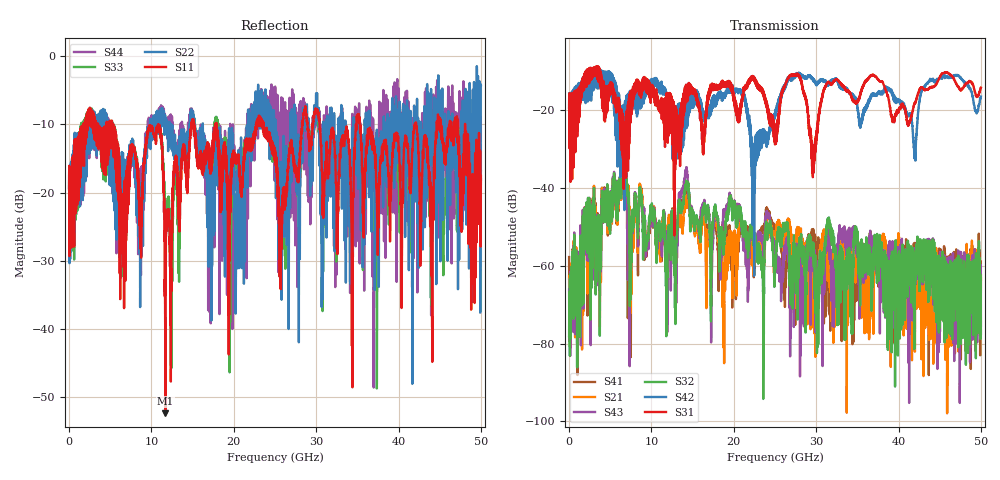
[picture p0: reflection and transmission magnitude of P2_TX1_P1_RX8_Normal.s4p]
!Keysight Technologies,N5225B,MY57041031,A.13.20.10
!Date: Friday, May 31, 2019 11:26:29
!Correction: S11(Full 4 Port(1,2,3,4))
!S12(Full 4 Port(1,2,3,4))
!S13(Full 4 Port(1,2,3,4))
!S14(Full 4 Port(1,2,3,4))
!S21(Full 4 Port(1,2,3,4))
!S22(Full 4 Port(1,2,3,4))
!S23(Full 4 Port(1,2,3,4))
!S24(Full 4 Port(1,2,3,4))
!S31(Full 4 Port(1,2,3,4))
!S32(Full 4 Port(1,2,3,4))
!S33(Full 4 Port(1,2,3,4))
!S34(Full 4 Port(1,2,3,4))
!S41(Full 4 Port(1,2,3,4))
!S42(Full 4 Port(1,2,3,4))
!S43(Full 4 Port(1,2,3,4))
!S44(Full 4 Port(1,2,3,4))
!S4P File: Measurements: <S11,S12,S13,S14>,
!<S21,S22,S23,S24>,
!<S31,S32,S33,S34>,
!<S41,S42,S43,S44>:
# Hz S  dB  R 50.0
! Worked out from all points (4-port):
!   5000 points, 10 MHz to 50 GHz, reference 50 ohm
!   strongest paths, dB at 10 MHz, 12.51 GHz, 25.01 GHz, 37.51 GHz, 50 GHz:
!     S31: -19.4, -17.3, -28.8, -12.1, -14.3
!     S42: -19.4, -24.1, -21.7, -15.8, -16.5
!     S32: -78.1, -46.9, -59.8, -54.8, -77.5
!     S43: -66.1, -47.3, -56.6, -58.4, -75.4
!     S21: -62.7, -46.6, -55.4, -57.9, -62.5
!     S41: -57.8, -46.8, -51.0, -61.0, -63.2
!   lowest |S11| = -52.3 dB at 11.69 GHz (marker M1), VSWR 1.00, Z = 49.8 - j0.14 ohm
!   |S11| at or under -10 dB: 5.36 GHz to 10.81 GHz (5.449 GHz wide, 67.4 % of centre); 17.89 GHz to 22.7 GHz (4.805 GHz wide, 23.7 % of centre); 35.31 GHz to 41.96 GHz (6.647 GHz wide, 17.2 % of centre)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
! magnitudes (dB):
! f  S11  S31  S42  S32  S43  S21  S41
! 10 MHz  -19.5  -19.4  -19.4  -78.1  -66.1  -62.7  -57.8
! 6.63 GHz  -30.9  -27.3  -26.3  -35.3  -35.7  -36.4  -36.7
! 7.34 GHz  -13.9  -17.4  -16.4  -56.9  -65.0  -50.7  -59.5
! 11.69 GHz  -52.3  -22.9  -16.1  -54.4  -51.0  -52.8  -51.7
! 22.38 GHz  -12.8  -11.4  -39.1  -54.5  -53.3  -60.4  -55.7
! 27.71 GHz  -16.9  -10.9  -10.8  -60.2  -57.2  -50.8  -60.2
! 50 GHz  -17.6  -14.3  -16.5  -77.5  -75.4  -62.5  -63.2
